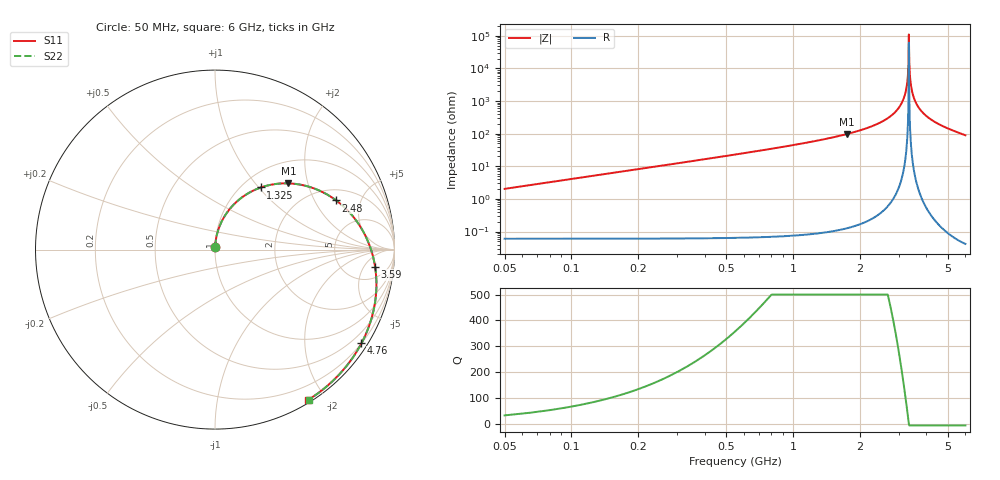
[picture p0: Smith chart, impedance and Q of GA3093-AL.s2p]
! Coilcraft GA3093-AL Air Core Inductor
! 01 July 2008
# MHZ S MA R 50
!Freq  MagS11  AngS11  MagS21  AngS21  MagS12  AngS12  MagS22  AngS22
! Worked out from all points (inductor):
!   398 points, 50 MHz to 6 GHz, reference 50 ohm
!   read as 1/Y11, port 2 shorted: L = 6.47 nH near 65 MHz
!   highest Q = 772 at 1.745 GHz (marker M1), where L = 8.8 nH
!   self-resonance near 3.335 GHz
!   S11 on the Smith chart (normalised r, x): 50 MHz: 1.00, +0.03; 1.325 GHz: 1.21, +1.03; 2.48 GHz: 2.60, +3.03; 3.59 GHz: 9, -9; 4.76 GHz: 0.20, -3.41; 6 GHz: 0.03, -1.80
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50  0.01679 86.6  0.9993 -1.4  0.9993 -1.4  0.01679 86.6
65  0.02181 86.6  0.9992 -1.8  0.9992 -1.8  0.02183 86.7
95  0.03187 86.3  0.9989 -2.6  0.9989 -2.6  0.03189 86.3
125  0.04193 85.8  0.9985 -3.4  0.9985 -3.4  0.04195 85.8
155  0.05199 85.1  0.998 -4.2  0.998 -4.2  0.05201 85.1
230  0.0771 83.3  0.9964 -6.3  0.9964 -6.3  0.07714 83.3
335  0.1122 80.5  0.9931 -9.2  0.9931 -9.2  0.1122 80.5
470  0.1571 76.9  0.987 -12.8  0.987 -12.8  0.1572 76.9
635  0.2115 72.5  0.9768 -17.4  0.9768 -17.4  0.2116 72.5
830  0.275 67.2  0.9608 -22.7  0.9608 -22.7  0.2751 67.2
1055  0.3467 61.0  0.9373 -28.9  0.9373 -28.9  0.3469 61.0
1325  0.4299 53.6  0.9022 -36.3  0.9022 -36.3  0.4301 53.6
1745  0.5509 42.1  0.8339 -47.9  0.8339 -47.9  0.5511 42.1
2045  0.6293 33.8  0.7765 -56.1  0.7765 -56.1  0.6296 33.8
2480  0.7285 22.1  0.6842 -67.9  0.6842 -67.9  0.7289 22.1
3035  0.828 7.6  0.56 -82.4  0.56 -82.4  0.8283 7.6
3590  0.8973 -6.2  0.4404 -96.2  0.4404 -96.2  0.8977 -6.2
4025  0.9337 -16.4  0.357 -106.4  0.357 -106.4  0.9341 -16.4
4760  0.9686 -32.6  0.2471 -122.6  0.2471 -122.6  0.969 -32.6
5015  0.9752 -38.0  0.2196 -128.0  0.2196 -128.0  0.9756 -38.0
5540  0.9831 -48.8  0.1812 -138.8  0.1812 -138.8  0.9834 -48.8
6000  0.9852 -58.1  0.1689 -148.1  0.1689 -148.1  0.9856 -58.1
